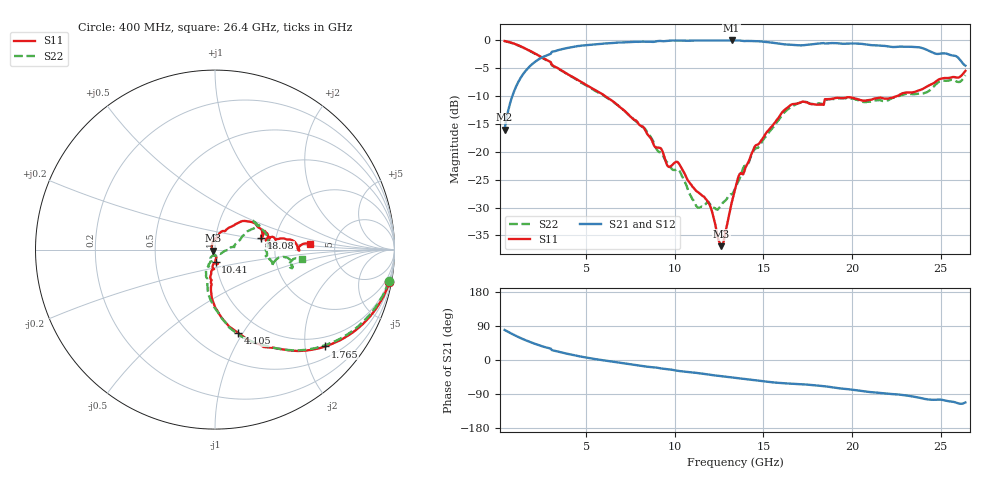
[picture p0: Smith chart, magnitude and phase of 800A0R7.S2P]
!  American Technical Ceramics  Date:  9/12/2007
!  One Norden Lane
!  Huntington Station,  NY.  11746-2102
!  Tel:  (631) 622-4700  Fax:  (631) 622-4748
!  Part Number  800A0R7  Mounting Orientation: Vertical
!  Description: Ultra Low ESR Microwave capacitors
!  Application: Coupling, Bypass, Tuning, DC Block
!  Filters, Matching
# GHZ S DB R 50
! Freq  |S11|  S11 Ph  |S21|  S21 Ph  |S12|  S12 Ph  |S22|  S22 Ph
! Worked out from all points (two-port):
!   401 points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, 400 MHz to 26.4 GHz, reference 50 ohm
!   highest |S21| = 0.00 dB at 13.21 GHz (marker M1); lowest = -16.0 dB at 400 MHz (marker M2)
!   |S21| within 3 dB of the highest: 2.545 GHz to 25.96 GHz (23.41 GHz wide, 164 % of centre)
!   lowest |S11| = -36.9 dB at 12.62 GHz (marker M3), VSWR 1.03, Z = 48.7 - j0.557 ohm
!   |S11| at or under -10 dB: 6.074 GHz to 22.53 GHz (16.46 GHz wide, 115 % of centre)
!   |S22| runs from -30.4 to -0.1 dB; largest |S21 - S12| = 0.0049
!   S11 on the Smith chart (normalised r, x): 400 MHz: 1, -11; 1.765 GHz: 0.75, -2.46; 4.105 GHz: 0.79, -0.96; 10.41 GHz: 1.00, -0.14; 18.08 GHz: 1.67, +0.24; 26.4 GHz: 3.26, +0.27
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0.4  -0.10 -10.7  -16.00 79.2  -16.01 79.2  -0.15 -10.3
0.985  -0.63 -25.2  -8.73 64.9  -8.73 64.9  -0.67 -24.6
1.765  -1.74 -41.3  -4.82 48.9  -4.84 48.8  -1.79 -40.8
3.195  -4.65 -64.7  -1.96 24.6  -1.97 24.6  -4.71 -64.3
4.105  -6.32 -74.4  -1.24 14.8  -1.25 14.8  -6.36 -75.5
4.755  -7.50 -80.7  -0.92 8.6  -0.92 8.7  -7.63 -81.0
8.2  -15.47 -97.3  -0.21 -16.2  -0.20 -16.1  -15.57 -105.3
9.11  -19.27 -92.5  -0.09 -21.2  -0.08 -21.1  -20.03 -110.3
9.63  -22.64 -88.4  -0.04 -24.3  -0.03 -24.2  -22.12 -110.7
10.41  -23.07 -87.1  -0.02 -29.9  -0.01 -29.9  -24.38 -115.7
11.32  -27.24 -79.2  -0.01 -34.6  -0.01 -34.6  -30.02 -99.5
11.97  -29.50 -92.9  -0.01 -38.9  -0.01 -38.9  -29.31 -80.8
12.62  -36.93 -156.3  -0.01 -42.5  -0.01 -42.5  -29.59 -51.0
13.205  -29.23 117.4  0.00 -45.9  -0.01 -45.9  -27.63 -26.9
13.4  -26.66 104.9  -0.01 -46.8  -0.01 -46.8  -26.64 -16.9
14.505  -19.09 68.3  -0.13 -52.8  -0.12 -52.9  -19.58 8.3
16.13  -12.65 43.1  -0.69 -61.2  -0.68 -61.3  -13.07 29.1
17.755  -11.43 16.3  -0.69 -65.9  -0.66 -66.0  -11.39 31.8
18.08  -11.54 14.6  -0.57 -67.6  -0.55 -67.7  -11.34 35.8
22.11  -10.38 11.3  -1.11 -89.6  -1.09 -89.8  -10.62 -7.5
23.8  -8.94 9.5  -1.24 -99.5  -1.23 -99.8  -9.55 -13.8
26.4  -5.47 3.2  -4.52 -112.1  -4.51 -112.2  -6.24 -6.3
